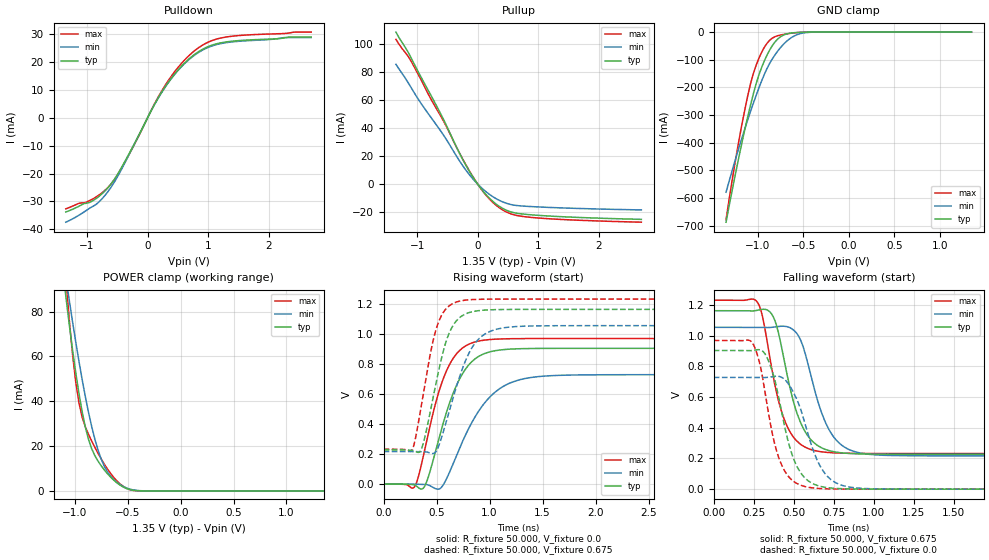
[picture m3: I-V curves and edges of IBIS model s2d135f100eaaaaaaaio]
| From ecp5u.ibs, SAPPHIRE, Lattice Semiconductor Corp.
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|   Model s2d135f100eaaaaaaaio
[Model] s2d135f100eaaaaaaaio
Model_type I/O
Polarity   Non-Inverting
Enable   Active-Low
Vinl =  0.575V
Vinh =  0.775V
Vmeas =  0.675V
Cref =  30.000pF
Rref =  50.000
Vref =  0.675V
C_comp   5.000pF   4.000pF   5.500pF
[Temperature Range]   25.000   0.125k   -40.000
[Voltage Range]   1.350V   1.280V   1.420V
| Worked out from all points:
|   slope of the pulldown table from 0 to 0.203 V, typ, clamps not added: 25.1 ohm
|   slope of the pullup table from 0 to 0.203 V, typ, clamps not added: 19.5 ohm
|   GND clamp passes 1 mA (typ) near -0.54 V on its own axis
|   POWER clamp passes 1 mA (typ) near -0.51 V on its own axis
|   rising waveform, R_fixture 50.000, V_fixture 0.0: 20-80 % time 259ps typ, 345ps min, 230ps max; typ from 0 V to 0.904 V
|   rising waveform, R_fixture 50.000, V_fixture 0.675: 20-80 % time 182ps typ, 238ps min, 161ps max; typ from 0.227 V to 1.16 V
|   falling waveform, R_fixture 50.000, V_fixture 0.675: 20-80 % time 137ps typ, 152ps min, 127ps max; typ from 1.16 V to 0.227 V
|   falling waveform, R_fixture 50.000, V_fixture 0.0: 20-80 % time 127ps typ, 148ps min, 113ps max; typ from 0.904 V to 0 V
[Pulldown]
|Voltage   I(typ)   I(min)   I(max)
-1.35V    -33.78mA   -37.41mA   -32.64mA
-850mV    -28.97mA   -31.05mA   -28.4mA
-600mV    -23.63mA   -24.79mA   -23.65mA
-350mV    -14.66mA   -15.1mA    -14.92mA
50mV      2.157mA    2.138mA    2.25mA
200mV     7.987mA    7.913mA    8.357mA
450mV     15.76mA    15.6mA     16.57mA
750mV     22.25mA    22mA       23.54mA
1V        25.47mA    25.19mA    27.06mA
1.3V      27.15mA    26.89mA    28.91mA
2.25V     28.55mA    28.68mA    30.15mA
2.7V      28.9mA     28.68mA    30.66mA
[Pullup]
|Voltage   I(typ)   I(min)   I(max)
-1.35V    108.6mA    85.6mA     103.4mA
-1.1V     90.26mA    69.04mA    87.95mA
-800mV    65.64mA    49.36mA    62.97mA
-600mV    49.28mA    37.29mA    47.89mA
-300mV    22.03mA    16.59mA    22.16mA
-150mV    10.08mA    7.445mA    10.4mA
100mV     -5.613mA   -4.06mA    -5.96mA
300mV     -14.08mA   -10.26mA   -14.96mA
550mV     -19.83mA   -14.55mA   -21.23mA
800mV     -21.55mA   -15.77mA   -23.33mA
1.5V      -23.43mA   -17.1mA    -25.43mA
2.7V      -25.1mA    -18.37mA   -27.13mA
[GND_clamp]
|Voltage   I(typ)   I(min)   I(max)
-1.35V    -687.3mA   -578.9mA   -678.1mA
-1.26V    -534.3mA   -475.1mA   -489.7mA
-1.2V     -438.1mA   -409.1mA   -376.7mA
-1.08V    -262.9mA   -286.2mA   -185.9mA
-1.02V    -187.7mA   -229.9mA   -120.7mA
-960mV    -129.1mA   -177.6mA   -73.95mA
-900mV    -83.6mA    -132.1mA   -40.76mA
-840mV    -48.57mA   -96.56mA   -21.66mA
-750mV    -16.65mA   -55.68mA   -10.64mA
-660mV    -4.958mA   -26.68mA   -5.448mA
-480mV    -317.7uA   -2.229mA   -341.9uA
1.35V     0A         0A         0A
[POWER_clamp]
|Voltage   I(typ)   I(min)   I(max)
-1.35V    211.5mA    193mA      324.9mA
-1.08V    85.33mA    94.25mA    92.93mA
-1.05V    73.76mA    84.65mA    75.65mA
-990mV    52.73mA    66.45mA    48.6mA
-960mV    43.53mA    57.9mA     39.38mA
-930mV    35.42mA    49.79mA    33mA
-840mV    18.88mA    28.82mA    22.31mA
-750mV    11.24mA    14.22mA    14.3mA
-660mV    6.13mA     6.499mA    7.742mA
-570mV    2.538mA    2.795mA    3.049mA
-390mV    57.41uA    134.8uA    35.81uA
1.35V     0A         0A         0A
[Ramp]
| variable   typ   min   max
dV/dt_r 0.542/0.260n   0.437/0.346n   0.581/0.233n
dV/dt_f 0.511/0.163n   0.485/0.173n   0.546/0.153n
R_load = 50.000
[Rising Waveform]
R_fixture= 50.000
V_fixture= 0.0
V_fixture_min= 0.0
V_fixture_max= 0.0
|time   V(typ)   V(min)   V(max)
0s        0V         0V         0V
286ps     -4.285mV   -438.7uV   -22.54mV
382ps     -20.1mV    -1.727mV   210.6mV
526ps     315.1mV    -31.84mV   625.3mV
627ps     549.6mV    87.38mV    802.5mV
774ps     766.8mV    328.9mV    919.7mV
944ps     866.2mV    532.4mV    957.4mV
1.214ns   898.9mV    678.7mV    967.5mV
1.653ns   903.3mV    723.7mV    968.6mV
10ns      903.5mV    728.2mV    968.6mV
[Rising Waveform]
R_fixture= 50.000
V_fixture= 0.675
V_fixture_min= 0.642
V_fixture_max= 0.710
|time   V(typ)   V(min)   V(max)
0s        227.4mV    216.8mV    232.4mV
261ps     225.4mV    216.7mV    221.5mV
347ps     219.8mV    215.7mV    486.9mV
454ps     531.1mV    203.3mV    914mV
524ps     770.2mV    261.8mV    1.088V
629ps     1.022V     510.2mV    1.191V
758ps     1.127V     795.7mV    1.223V
954ps     1.158V     997.7mV    1.23V
1.324ns   1.162V     1.051V     1.231V
10ns      1.163V     1.054V     1.231V
[Falling Waveform]
R_fixture= 50.000
V_fixture= 0.675
V_fixture_min= 0.642
V_fixture_max= 0.710
|time   V(typ)   V(min)   V(max)
0s        1.163V     1.054V     1.231V
265ps     1.164V     1.055V     1.227V
303ps     1.171V     1.054V     1.132V
359ps     1.145V     1.054V     806.1mV
432ps     883.1mV    1.062V     479.9mV
531ps     464.7mV    996mV      302.3mV
701ps     257.5mV    428.7mV    240mV
842ps     232.9mV    259.8mV    233.6mV
1.112ns   227.7mV    219.2mV    232.4mV
10ns      227.4mV    216.8mV    232.4mV
[Falling Waveform]
R_fixture= 50.000
V_fixture= 0.0
V_fixture_min= 0.0
V_fixture_max= 0.0
|time   V(typ)   V(min)   V(max)
0s        903.5mV    728.2mV    968.6mV
232ps     902.3mV    728.2mV    963.7mV
317ps     886.6mV    727.1mV    654.5mV
372ps     747.3mV    734.3mV    334mV
432ps     461.7mV    724mV      140.6mV
522ps     143.7mV    578.2mV    35.77mV
633ps     29.57mV    222.5mV    6.677mV
754ps     5.437mV    46.81mV    1.146mV
1.003ns   267.6uV    2.198mV    49.35uV
10ns      0V         0V         0V
